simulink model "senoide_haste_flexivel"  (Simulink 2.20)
settings: Solver=ode1  StartTime=0.0  StopTime=50  FixedStep=0.001  RelTol=1e-3  AbsTol=1e-6
libraries: winlib x4

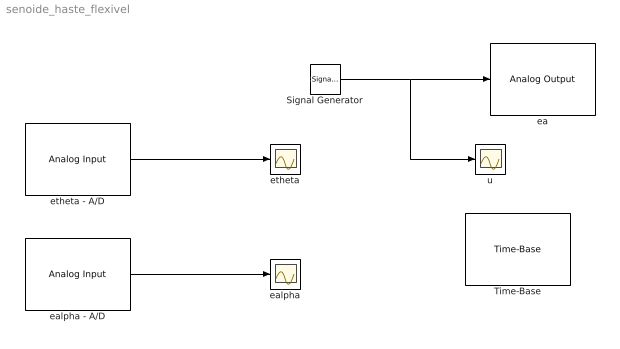
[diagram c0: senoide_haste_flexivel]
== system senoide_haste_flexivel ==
  Signal Generator : SignalGenerator  WaveForm=sine  Amplitude=1  Frequency=1.4415  Units=Hertz
  Time-Base : winlib/Quanser Consulting MultiQ Series/Time-Base  baseAddr=0x320  irqLevel=9  clockSource=1
  ea : winlib/Quanser Consulting MultiQ Series/Analog Output  baseAddr=0x320  channels=[4]  initialOutputs=0  finalOutputs=0  sampleTime=str2num(get_param(bdroot, 'FixedStep'))
  ealpha : Scope
  ealpha - A/D : winlib/Quanser Consulting MultiQ Series/Analog Input  baseAddr=0x320  channels=[2]  sampleTime=str2num(get_param(bdroot, 'FixedStep'))
  etheta : Scope
  etheta - A/D : winlib/Quanser Consulting MultiQ Series/Analog Input  baseAddr=0x320  channels=[1]  sampleTime=str2num(get_param(bdroot, 'FixedStep'))
  u : Scope
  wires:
  etheta - A/D/1 -> etheta/1
  Signal Generator/1 -> ea/1, u/1
  ealpha - A/D/1 -> ealpha/1
